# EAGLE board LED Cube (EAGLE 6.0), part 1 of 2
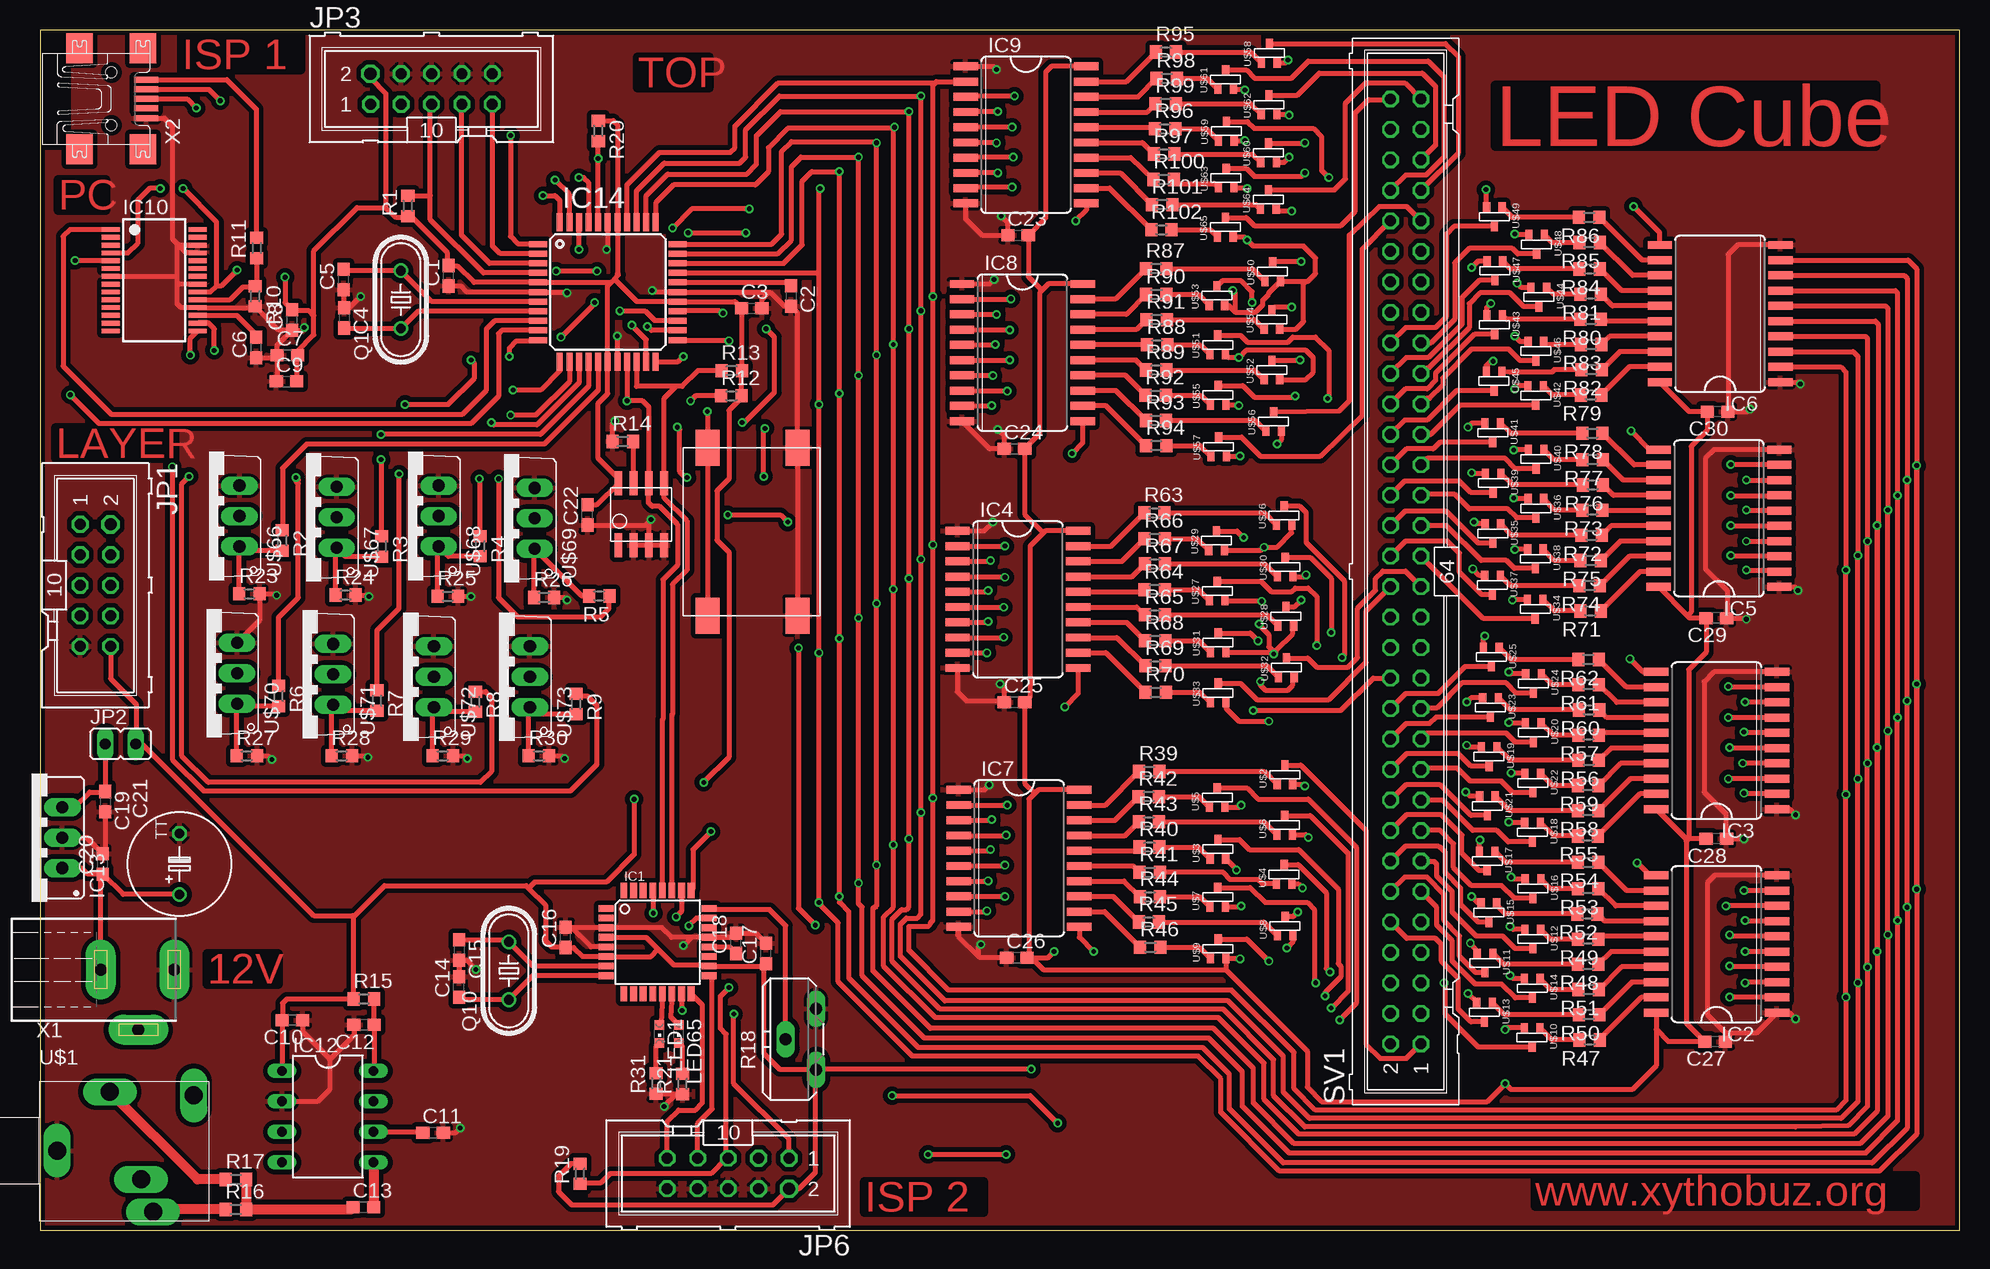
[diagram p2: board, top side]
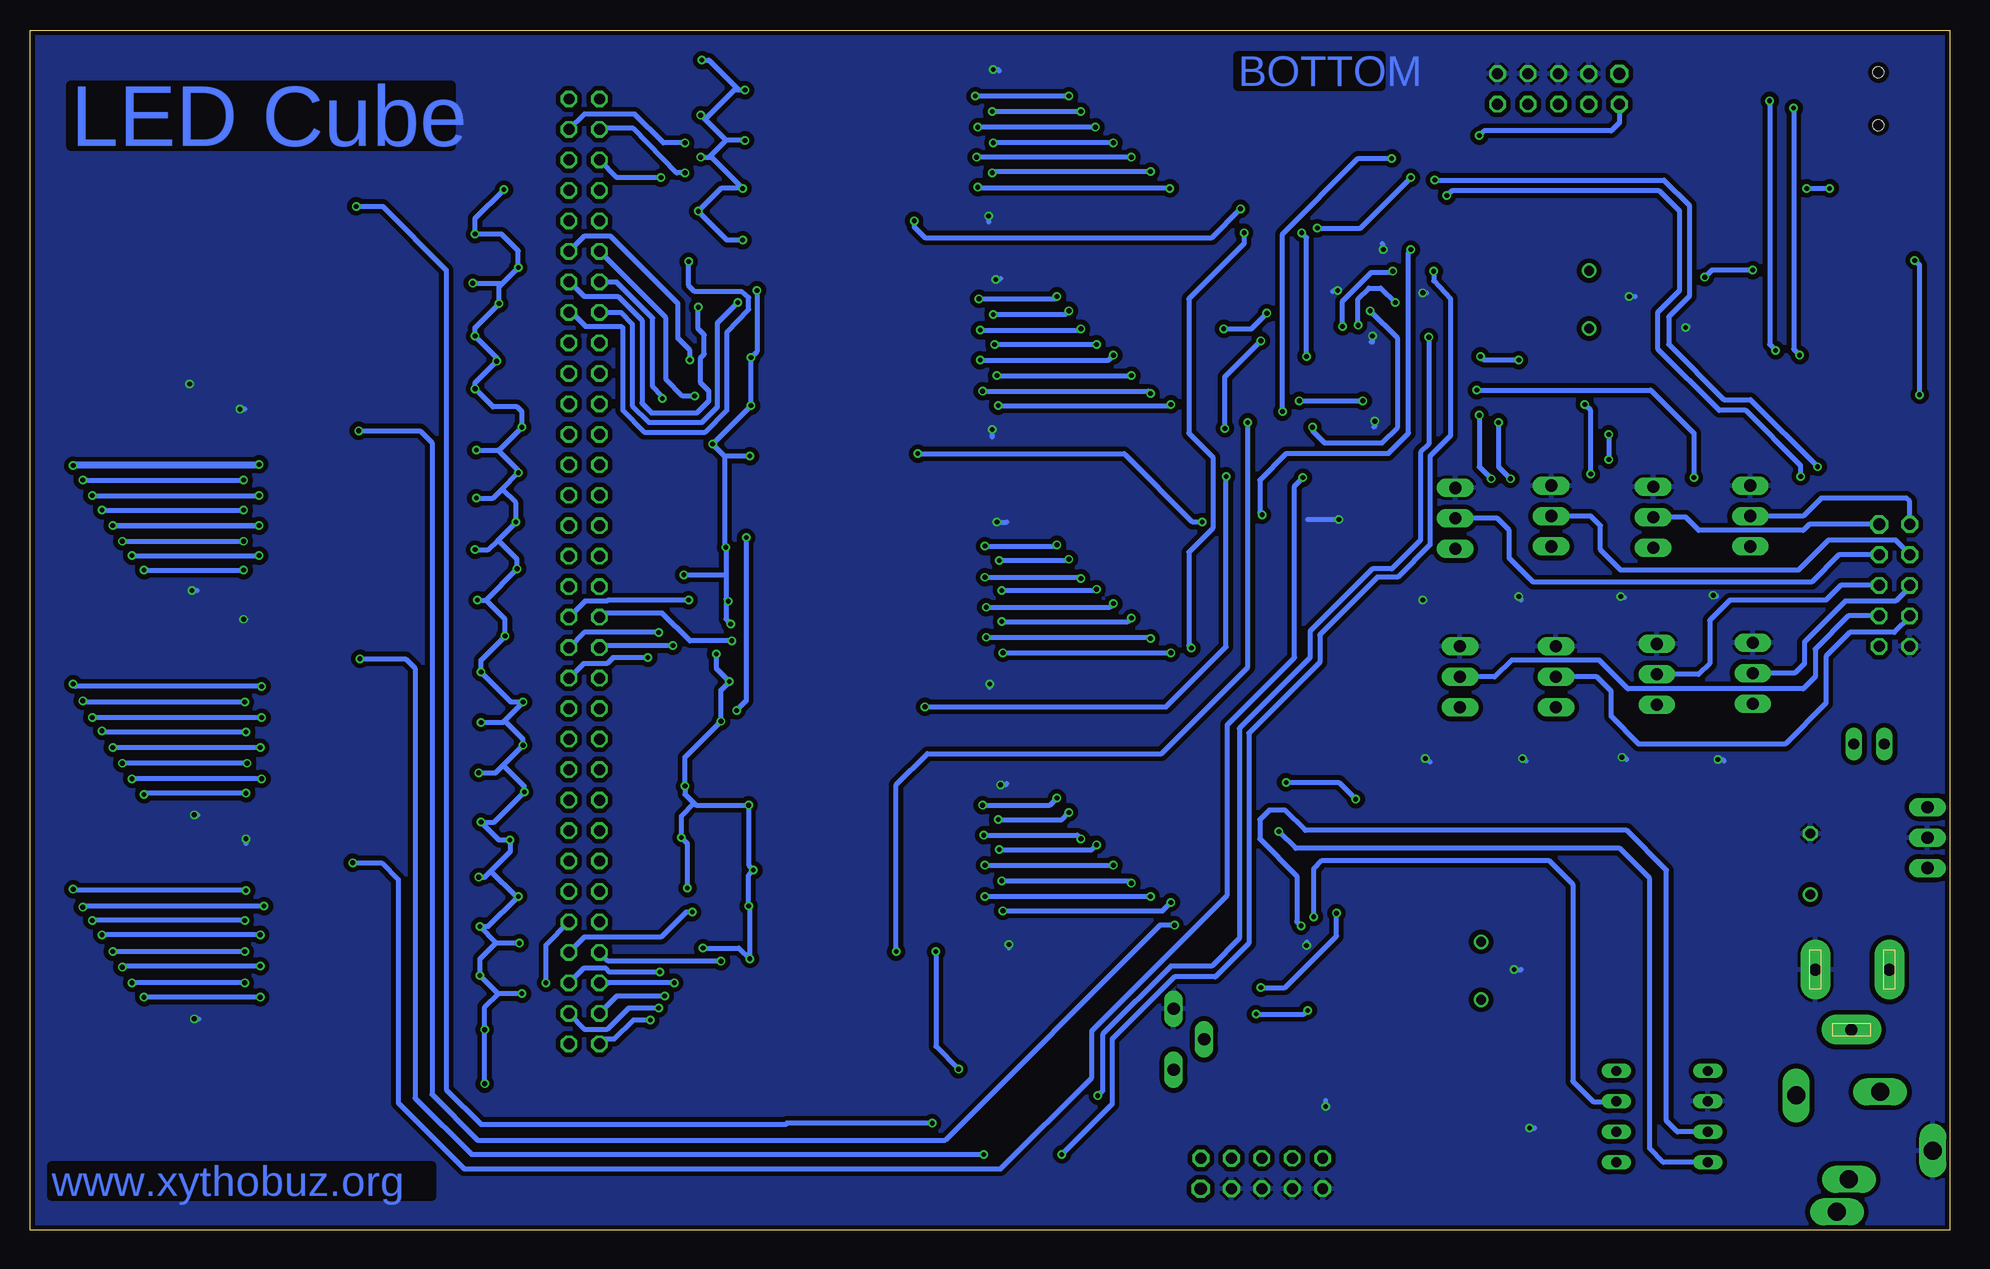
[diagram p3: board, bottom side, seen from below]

Size 160 x 100 mm. Coordinates in mm from the lower left corner, seen from the top.
Outline: 0,0 160,0 160,100 0,100 0,0
Copper layers (1*16): Top 0.035mm / dielectric 1.5mm / Bottom 0.035mm
Design rules: minimum track width 0.15mm, minimum drill 0.3mm, track to track 0.15mm, track to pad 0.15mm, pad to pad 0.15mm, via to via 0.15mm, smd to smd 0.1mm, copper to edge 0.15mm, drill to drill 0.15mm, minimum pad ring 0.15mm, minimum via ring 0.15mm, stop-mask expansion 4mil, vias tented up to drill 0mil, thermal gap 10mil

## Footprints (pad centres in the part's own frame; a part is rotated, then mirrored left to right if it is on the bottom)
C0603 = smd 1.1 x 1: 1 -0.85,0; 2 0.85,0
TAP5-80 = drill 0.813: + -2.54,0 | drill 0.813 octagon: - 2.54,0
TQFP32-08 = smd 1.27 x 0.559: 1 -4.293,2.8; 2 -4.293,2; 3 -4.293,1.2; 4 -4.293,0.4; 5 -4.293,-0.4; 6 -4.293,-1.2; 7 -4.293,-2; 8 -4.293,-2.8; 17 4.293,-2.8; 18 4.293,-2; 19 4.293,-1.2; 20 4.293,-0.4; 21 4.293,0.4; 22 4.293,1.2; 23 4.293,2; 24 4.293,2.8 | smd 0.559 x 1.27: 9 -2.8,-4.293; 10 -2,-4.293; 11 -1.2,-4.293; 12 -0.4,-4.293; 13 0.4,-4.293; 14 1.2,-4.293; 15 2,-4.293; 16 2.8,-4.293; 25 2.8,4.293; 26 2,4.293; 27 1.2,4.293; 28 0.4,4.293; 29 -0.4,4.293; 30 -1.2,4.293; 31 -2,4.293; 32 -2.8,4.293
SO20W = smd 0.66 x 2.032: 1 -5.715,-5.029; 2 -4.445,-5.029; 3 -3.175,-5.029; 4 -1.905,-5.029; 5 -0.635,-5.029; 6 0.635,-5.029; 7 1.905,-5.029; 8 3.175,-5.029; 9 4.445,-5.029; 10 5.715,-5.029; 11 5.715,5.029; 12 4.445,5.029; 13 3.175,5.029; 14 1.905,5.029; 15 0.635,5.029; 16 -0.635,5.029; 17 -1.905,5.029; 18 -3.175,5.029; 19 -4.445,5.029; 20 -5.715,5.029
SSOP28 = smd 0.4 x 1.5: 1 -4.225,-3.625; 2 -3.575,-3.625; 3 -2.925,-3.625; 4 -2.275,-3.625; 5 -1.625,-3.625; 6 -0.975,-3.625; 7 -0.325,-3.625; 8 0.325,-3.625; 9 0.975,-3.625; 10 1.625,-3.625; 11 2.275,-3.625; 12 2.925,-3.625; 13 3.575,-3.625; 14 4.225,-3.625; 15 4.225,3.625; 16 3.575,3.625; 17 2.925,3.625; 18 2.275,3.625; 19 1.625,3.625; 20 0.975,3.625; 21 0.325,3.625; 22 -0.325,3.625; 23 -0.975,3.625; 24 -1.625,3.625; 25 -2.275,3.625; 26 -2.925,3.625; 27 -3.575,3.625; 28 -4.225,3.625
SOIC8 = smd 0.65 x 2: PA 0.635,-1; PB 1.905,-1; PC 3.175,-1; PD 4.445,-1; PE 4.445,4.2; PF 3.175,4.2; PG 1.905,4.2; PH 0.635,4.2
DIP8 = drill 0.813 long: 1 -3.81,-3.81; 2 -1.27,-3.81; 3 1.27,-3.81; 4 3.81,-3.81; 5 3.81,3.81; 6 1.27,3.81; 7 -1.27,3.81; 8 -3.81,3.81
78XXS = drill 1.016 long: GND 0,-2.54; IN -2.54,-2.54; OUT 2.54,-2.54
TQFP44 = smd 1.5 x 0.5: 1 -5.8,4; 2 -5.8,3.2; 3 -5.8,2.4; 4 -5.8,1.6; 5 -5.8,0.8; 6 -5.8,0; 7 -5.8,-0.8; 8 -5.8,-1.6; 9 -5.8,-2.4; 10 -5.8,-3.2; 11 -5.8,-4; 23 5.8,-4; 24 5.8,-3.2; 25 5.8,-2.4; 26 5.8,-1.6; 27 5.8,-0.8; 28 5.8,0; 29 5.8,0.8; 30 5.8,1.6; 31 5.8,2.4; 32 5.8,3.2; 33 5.8,4 | smd 0.5 x 1.5: 12 -4,-5.8; 13 -3.2,-5.8; 14 -2.4,-5.8; 15 -1.6,-5.8; 16 -0.8,-5.8; 17 0,-5.8; 18 0.8,-5.8; 19 1.6,-5.8; 20 2.4,-5.8; 21 3.2,-5.8; 22 4,-5.8; 34 4,5.8; 35 3.2,5.8; 36 2.4,5.8; 37 1.6,5.8; 38 0.8,5.8; 39 0,5.8; 40 -0.8,5.8; 41 -1.6,5.8; 42 -2.4,5.8; 43 -3.2,5.8; 44 -4,5.8
ML10 = drill 0.914 pad 1.422 octagon: 1 -5.08,-1.27; 3 -2.54,-1.27; 4 -2.54,1.27 | drill 1.016 pad 1.422 octagon: 2 -5.08,1.27 | drill 0.914 octagon: 5 0,-1.27; 6 0,1.27; 7 2.54,-1.27; 8 2.54,1.27; 9 5.08,-1.27; 10 5.08,1.27
JP1 = drill 0.914 long: 1 0,-1.27; 2 0,1.27
CHIPLED_0603 = smd 0.8 x 0.8: A 0,-0.75; C 0,0.75
HC49/S = drill 0.813: 1 -2.413,0; 2 2.413,0
R0603 = smd 1 x 1.1: 1 -0.85,0; 2 0.85,0
PT-10S = drill 1.016 long: A -2.54,-1.27; E 2.54,-1.27; S 0,1.27
ML64 = drill 0.914 octagon: 1 -39.37,-1.27; 2 -39.37,1.27; 3 -36.83,-1.27; 4 -36.83,1.27; 5 -34.29,-1.27; 6 -34.29,1.27; 7 -31.75,-1.27; 8 -31.75,1.27; 9 -29.21,-1.27; 10 -29.21,1.27; 11 -26.67,-1.27; 12 -26.67,1.27; 13 -24.13,-1.27; 14 -24.13,1.27; 15 -21.59,-1.27; 16 -21.59,1.27; 17 -19.05,-1.27; 18 -19.05,1.27; 19 -16.51,-1.27; 20 -16.51,1.27; 21 -13.97,-1.27; 22 -13.97,1.27; 23 -11.43,-1.27; 24 -11.43,1.27; 25 -8.89,-1.27; 26 -8.89,1.27; 27 -6.35,-1.27; 28 -6.35,1.27; 29 -3.81,-1.27; 30 -3.81,1.27; 31 -1.27,-1.27; 32 -1.27,1.27; 33 1.27,-1.27; 34 1.27,1.27; 35 3.81,-1.27; 36 3.81,1.27; 37 6.35,-1.27; 38 6.35,1.27; 39 8.89,-1.27; 40 8.89,1.27; 41 11.43,-1.27; 42 11.43,1.27; 43 13.97,-1.27; 44 13.97,1.27; 45 16.51,-1.27; 46 16.51,1.27; 47 19.05,-1.27; 48 19.05,1.27; 49 21.59,-1.27; 50 21.59,1.27; 51 24.13,-1.27; 52 24.13,1.27; 53 26.67,-1.27; 54 26.67,1.27; 55 29.21,-1.27; 56 29.21,1.27; 57 31.75,-1.27; 58 31.75,1.27; 59 34.29,-1.27; 60 34.29,1.27; 61 36.83,-1.27; 62 36.83,1.27; 63 39.37,-1.27; 64 39.37,1.27
KLINKEPRINT = drill 1.5 pad 1.778 long: CONLEFT 12.9,10.45; CONRIGHT 8.5,3.45; GND 1.5,5.85; LEFT 5.9,10.75; RIGHT 9.5,0.75
SOT323 = smd 0.6 x 0.8: P$1 -0.65,-0.65; P$2 0.65,-0.65; P$3 0,0.95
TO220-3V = drill 1.016 long: 1 -2.54,0; 2 0,0; 3 2.54,0
SMDTASTER = smd 3 x 2: A 0,7.5; A2 14,7.5; B 0,0; B2 14,0
733980-62 = drill 1 pad 2.5 long: 1 0,8.57; 2 0,2.42; 3 5,5.57
USB-B-MINI-SMD = smd 2 x 0.5: 1 2.9,1.6; 2 2.9,0.8; 3 2.9,0; 4 2.9,-0.8; 5 2.9,-1.6 | smd 2.2 x 2.5: M1 -2.65,-4.2; M2 -2.65,4.2; M3 2.65,4.2; M4 2.65,-4.2 | hole 0.9: 0,2.2; 0,-2.2

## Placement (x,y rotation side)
C1  100n  [C0603]  34.04,79.52 90 top
C2  100n  [C0603]  62.56,77.83 270 top
C3  100n  [C0603]  59.29,76.81 0 top
C4  22p  [C0603]  25.31,76.01 270 top
C5  22p  [C0603]  25.29,79.21 90 top
C6  100n  [C0603]  17.99,73.54 90 top
C7  100n  [C0603]  20.59,72.91 0 top
C8  100n  [C0603]  20.99,75.84 90 top
C9  4u7  [C0603]  20.53,70.71 0 top
C10  100n  [C0603]  21.01,17.49 180 top
C11  100n  [C0603]  32.74,8.11 0 top
C12  33p  [C0603]  26.99,17.09 180 top
C13  10n  [C0603]  26.93,1.91 0 top
C14  12p  [C0603]  34.89,20.25 90 top
C15  12p  [C0603]  34.91,23.33 270 top
C16  100n  [C0603]  43.79,24.39 90 top
C17  100n  [C0603]  60.49,23.04 90 top
C18  100n  [C0603]  57.99,23.89 90 top
C19  [C0603]  5.4,35.7 270 top
C20  [C0603]  5.2,30.5 90 top
C21  [TAP5-80]  11.6,30.5 90 top
C22  [C0603]  45.6,59.6 90 top
C23  [C0603]  81.5,82.9 0 top
C24  [C0603]  81.2,65.1 0 top
C25  [C0603]  81.2,44 0 top
C26  [C0603]  81.4,22.7 0 top
C27  [C0603]  139.6,15.7 180 top
C28  [C0603]  139.7,32.6 180 top
C29  [C0603]  139.7,51 180 top
C30  [C0603]  139.8,68.2 180 top
IC1  MEGA8-AI  [TQFP32-08]  51.45,23.99 0 top
IC2  74HC573D  [SO20W]  139.72,23.83 90 top
IC3  74HC573D  [SO20W]  139.72,40.79 90 top
IC4  74HC573D  [SO20W]  81.48,52.55 270 top
IC5  74HC573D  [SO20W]  139.92,59.31 90 top
IC6  74HC573D  [SO20W]  140.02,76.37 90 top
IC7  74HC573D  [SO20W]  81.58,30.97 270 top
IC8  74HC573D  [SO20W]  81.86,73.12 270 top
IC9  74HC573D  [SO20W]  82.16,91.26 270 top
IC10  FT232RL  [SSOP28]  9.49,79.15 270 top
IC11  FM24V10  [SOIC8]  47.55,58.05 0 top
IC12  MSGEQ7  [DIP8]  23.96,9.45 270 top
IC13  [78XXS]  -0.7,32.7 90 top
IC14  MEGA32-A  [TQFP44]  47.3,78.16 0 top
JP1  [ML10]  4.59,53.72 270 top
JP2  [JP1]  6.7,40.5 270 top
JP3  AVR-ISP  [ML10]  32.6,95.09 0 top
JP6  AVR-ISP  [ML10]  57.33,4.71 180 top
LED1  [CHIPLED_0603]  51.6,16.35 180 top
LED65  [CHIPLED_0603]  53.22,16.35 180 top
Q1  [HC49/S]  30.05,77.53 90 top
Q10  [HC49/S]  39.05,21.6 90 top
R1  10k  [R0603]  30.64,85.35 90 top
R2  15  [R0603]  20.16,57.46 270 top
R3  15  [R0603]  28.46,56.97 270 top
R4  15  [R0603]  36.66,56.98 270 top
R5  15  [R0603]  46.59,52.84 180 top
R6  15  [R0603]  19.86,44.5 270 top
R7  15  [R0603]  28.06,44.11 270 top
R8  15  [R0603]  36.26,44.02 270 top
R9  15  [R0603]  44.66,43.83 270 top
R10  10k  [R0603]  17.91,77.81 270 top
R11  4k7  [R0603]  18.04,81.83 90 top
R12  2k  [R0603]  57.61,69.51 0 top
R13  2k  [R0603]  57.63,71.61 0 top
R14  1k  [R0603]  48.55,65.71 0 top
R15  200k  [R0603]  26.97,19.25 0 top
R16  200k  [R0603]  16.29,1.71 0 top
R17  200k  [R0603]  16.31,4.21 0 top
R18  [PT-10S]  63.4,15.9 90 top
R19  10k  [R0603]  44.99,4.69 90 top
R20  1k  [R0603]  46.51,91.59 270 top
R21  1k  [R0603]  53.53,12.18 90 top
R23  100k  [R0603]  17.43,53.01 0 top
R24  100k  [R0603]  25.45,52.91 0 top
R25  100k  [R0603]  33.97,52.81 0 top
R26  100k  [R0603]  41.99,52.71 0 top
R27  100k  [R0603]  17.21,39.51 0 top
R28  100k  [R0603]  25.13,39.51 0 top
R29  100k  [R0603]  33.55,39.51 0 top
R30  100k  [R0603]  41.57,39.51 0 top
R31  1k  [R0603]  51.33,12.22 90 top
R39  1k  [R0603]  92.43,38.21 0 top
R40  1k  [R0603]  92.45,31.91 0 top
R41  1k  [R0603]  92.47,29.81 0 top
R42  1k  [R0603]  92.39,36.11 0 top
R43  1k  [R0603]  92.41,34.01 0 top
R44  1k  [R0603]  92.49,27.76 0 top
R45  1k  [R0603]  92.41,25.66 0 top
R46  1k  [R0603]  92.53,23.56 0 top
R47  1k  [R0603]  129.15,15.84 180 top
R48  1k  [R0603]  129.03,22.14 180 top
R49  1k  [R0603]  129.01,24.24 180 top
R50  1k  [R0603]  129.09,17.94 180 top
R51  1k  [R0603]  129.07,20.04 180 top
R52  1k  [R0603]  128.95,26.34 180 top
R53  1k  [R0603]  129.03,28.44 180 top
R54  1k  [R0603]  129.01,30.64 180 top
R55  1k  [R0603]  128.99,32.84 180 top
R56  1k  [R0603]  129.07,39.14 180 top
R57  1k  [R0603]  129.05,41.24 180 top
R58  1k  [R0603]  129.03,34.94 180 top
R59  1k  [R0603]  129.01,37.04 180 top
R60  1k  [R0603]  129.09,43.34 180 top
R61  1k  [R0603]  129.07,45.44 180 top
R62  1k  [R0603]  129.05,47.54 180 top
R63  1k  [R0603]  92.87,59.76 0 top
R64  1k  [R0603]  92.89,53.36 0 top
R65  1k  [R0603]  92.91,51.26 0 top
R66  1k  [R0603]  92.89,57.61 0 top
R67  1k  [R0603]  92.91,55.51 0 top
R68  1k  [R0603]  92.93,49.11 0 top
R69  1k  [R0603]  92.95,47.01 0 top
R70  1k  [R0603]  92.97,44.81 0 top
R71  1k  [R0603]  129.21,51.59 180 top
R72  1k  [R0603]  129.29,57.89 180 top
R73  1k  [R0603]  129.37,59.99 180 top
R74  1k  [R0603]  129.15,53.69 180 top
R75  1k  [R0603]  129.23,55.79 180 top
R76  1k  [R0603]  129.41,62.09 180 top
R77  1k  [R0603]  129.39,64.19 180 top
R78  1k  [R0603]  129.37,66.39 180 top
R79  1k  [R0603]  129.25,69.59 180 top
R80  1k  [R0603]  129.23,75.89 180 top
R81  1k  [R0603]  129.21,77.99 180 top
R82  1k  [R0603]  129.29,71.69 180 top
R83  1k  [R0603]  129.27,73.79 180 top
R84  1k  [R0603]  129.15,80.09 180 top
R85  1k  [R0603]  129.13,82.29 180 top
R86  1k  [R0603]  129.11,84.39 180 top
R87  1k  [R0603]  93.01,80.11 0 top
R88  1k  [R0603]  93.09,73.76 0 top
R89  1k  [R0603]  93.01,71.66 0 top
R90  1k  [R0603]  93.03,77.96 0 top
R91  1k  [R0603]  93.05,75.86 0 top
R92  1k  [R0603]  92.97,69.56 0 top
R93  1k  [R0603]  92.99,67.46 0 top
R94  1k  [R0603]  93.01,65.36 0 top
R95  1k  [R0603]  93.83,98.16 0 top
R96  1k  [R0603]  93.75,91.76 0 top
R97  1k  [R0603]  93.67,89.66 0 top
R98  1k  [R0603]  93.89,95.96 0 top
R99  1k  [R0603]  93.81,93.86 0 top
R100  1k  [R0603]  93.65,87.55 0 top
R101  1k  [R0603]  93.5,85.45 0 top
R102  1k  [R0603]  93.45,83.35 0 top
SV1  [ML64]  113.81,54.88 90 top
U$1  KLINKENBUCHSE  [KLINKEPRINT]  -0.11,0.77 0 top
U$2  PNP  [SOT323]  103.74,37.79 0 top
U$3  PNP  [SOT323]  98.16,31.59 0 top
U$4  PNP  [SOT323]  103.68,29.49 0 top
U$5  PNP  [SOT323]  98.1,35.89 0 top
U$6  PNP  [SOT323]  103.72,33.59 0 top
U$7  PNP  [SOT323]  98.14,27.59 0 top
U$8  PNP  [SOT323]  103.76,25.19 0 top
U$9  PNP  [SOT323]  98.18,23.29 0 top
U$10  PNP  [SOT323]  124.34,16.2 180 top
U$11  PNP  [SOT323]  120.42,22.4 180 top
U$12  PNP  [SOT323]  124.4,24.4 180 top
U$13  PNP  [SOT323]  120.38,18.3 180 top
U$14  PNP  [SOT323]  124.36,20.3 180 top
U$15  PNP  [SOT323]  120.74,26.6 180 top
U$16  PNP  [SOT323]  124.42,28.6 180 top
U$17  PNP  [SOT323]  120.6,30.9 180 top
U$18  PNP  [SOT323]  124.38,33.3 180 top
U$19  PNP  [SOT323]  120.76,39.6 180 top
U$20  PNP  [SOT323]  124.44,41.6 180 top
U$21  PNP  [SOT323]  120.62,35.5 180 top
U$22  PNP  [SOT323]  124.4,37.4 180 top
U$23  PNP  [SOT323]  120.88,43.7 180 top
U$24  PNP  [SOT323]  124.46,45.7 180 top
U$25  PNP  [SOT323]  120.94,47.9 180 top
U$26  PNP  [SOT323]  103.68,59.4 0 top
U$27  PNP  [SOT323]  98.1,53.1 0 top
U$28  PNP  [SOT323]  103.82,51 0 top
U$29  PNP  [SOT323]  98.04,57.3 0 top
U$30  PNP  [SOT323]  103.76,55.1 0 top
U$31  PNP  [SOT323]  98.18,48.8 0 top
U$32  PNP  [SOT323]  103.86,46.71 0 top
U$33  PNP  [SOT323]  98.18,44.61 0 top
U$34  PNP  [SOT323]  124.6,51.89 180 top
U$35  PNP  [SOT323]  121.08,58.19 180 top
U$36  PNP  [SOT323]  124.66,60.29 180 top
U$37  PNP  [SOT323]  121.04,53.89 180 top
U$38  PNP  [SOT323]  124.62,56.09 180 top
U$39  PNP  [SOT323]  121.1,62.39 180 top
U$40  PNP  [SOT323]  124.68,64.39 180 top
U$41  PNP  [SOT323]  121.06,66.59 180 top
U$42  PNP  [SOT323]  124.64,69.69 180 top
U$43  PNP  [SOT323]  121.22,75.59 180 top
U$44  PNP  [SOT323]  124.9,77.89 180 top
U$45  PNP  [SOT323]  121.18,70.89 180 top
U$46  PNP  [SOT323]  124.66,73.39 180 top
U$47  PNP  [SOT323]  121.24,80.09 180 top
U$48  PNP  [SOT323]  124.72,82.29 180 top
U$49  PNP  [SOT323]  121.2,84.59 180 top
U$50  PNP  [SOT323]  102.72,79.71 0 top
U$51  PNP  [SOT323]  98.14,73.61 0 top
U$52  PNP  [SOT323]  102.66,71.51 0 top
U$53  PNP  [SOT323]  98.08,77.71 0 top
U$54  PNP  [SOT323]  102.66,75.72 0 top
U$55  PNP  [SOT323]  98.18,69.42 0 top
U$56  PNP  [SOT323]  102.8,67.22 0 top
U$57  PNP  [SOT323]  98.22,65.12 0 top
U$58  PNP  [SOT323]  102.44,97.92 0 top
U$59  PNP  [SOT323]  98.86,91.42 0 top
U$60  PNP  [SOT323]  102.38,89.62 0 top
U$61  PNP  [SOT323]  98.8,95.72 0 top
U$62  PNP  [SOT323]  102.42,93.62 0 top
U$63  PNP  [SOT323]  98.84,87.52 0 top
U$64  PNP  [SOT323]  102.36,85.72 0 top
U$65  PNP  [SOT323]  98.78,83.42 0 top
U$66  IRF530  [TO220-3V]  16.6,59.5 90 top
U$67  IRF530  [TO220-3V]  24.7,59.4 90 top
U$68  IRF530  [TO220-3V]  33.2,59.5 90 top
U$69  IRF530  [TO220-3V]  41.2,59.3 90 top
U$70  IRF530  [TO220-3V]  16.4,46.4 90 top
U$71  IRF530  [TO220-3V]  24.4,46.3 90 top
U$72  IRF530  [TO220-3V]  32.8,46.1 90 top
U$73  IRF530  [TO220-3V]  40.8,46.1 90 top
U$74  TASTER  [SMDTASTER]  63.1,51.2 90 top
X1  [733980-62]  2.6,21.7 270 top
X2  [USB-B-MINI-SMD]  5.92,94.26 0 top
